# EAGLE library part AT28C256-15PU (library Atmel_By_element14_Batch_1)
Paged Parallel EEPROM
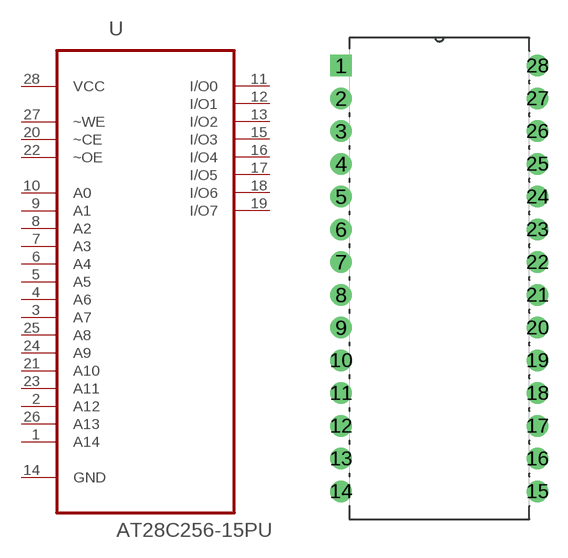
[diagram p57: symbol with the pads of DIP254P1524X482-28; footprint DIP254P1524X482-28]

Designator prefix U

## AT28C256-15PU (DESCRIPTION: Paged Parallel EEPROM; MPN: AT28C256-15PU; OC_FARNELL: 1095782; OC_NEWARK: 96K6555; PACKAGE: PDIP-28; SUPPLIER: ATMEL)  [DIP254P1524X482-28]
1  A14  in
2  A12  in
3  A7  in
4  A6  in
5  A5  in
6  A4  in
7  A3  in
8  A2  in
9  A1  in
10  A0  in
11  I/O0
12  I/O1
13  I/O2
14  GND  pas
15  I/O3
16  I/O4
17  I/O5
18  I/O6
19  I/O7
20  ~CE  in
21  A10  in
22  ~OE  in
23  A11  in
24  A9  in
25  A8  in
26  A13  in
27  ~WE  in
28  VCC  pwr

## Footprint DIP254P1524X482-28 (pad centres in mm)
drill 1.118 square: 1 -15.24,33.02
drill 1.118: 2 -15.24,30.48; 3 -15.24,27.94; 4 -15.24,25.4; 5 -15.24,22.86; 6 -15.24,20.32; 7 -15.24,17.78; 8 -15.24,15.24; 9 -15.24,12.7; 10 -15.24,10.16; 11 -15.24,7.62; 12 -15.24,5.08; 13 -15.24,2.54; 14 -15.24,0; 15 0,0; 16 0,2.54; 17 0,5.08; 18 0,7.62; 19 0,10.16; 20 0,12.7; 21 0,15.24; 22 0,17.78; 23 0,20.32; 24 0,22.86; 25 0,25.4; 26 0,27.94; 27 0,30.48; 28 0,33.02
